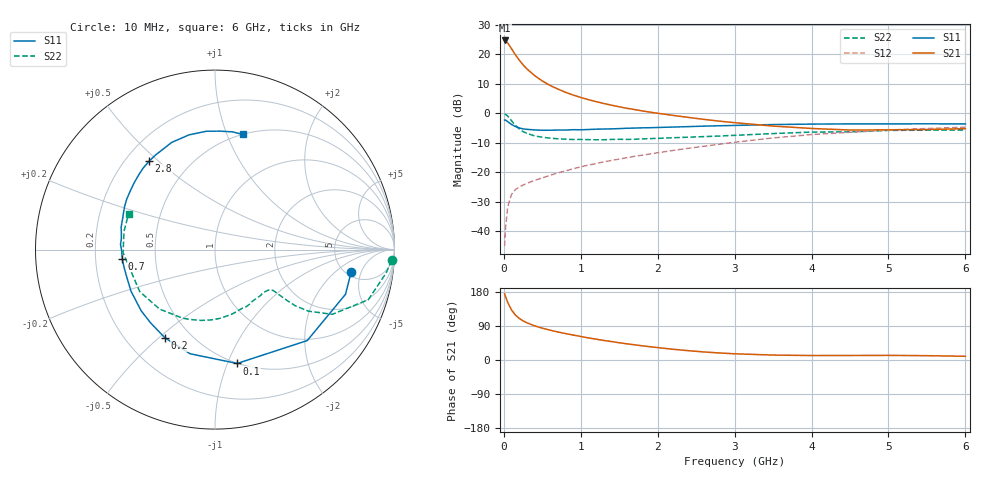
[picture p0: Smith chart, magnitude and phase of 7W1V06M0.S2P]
! Infineon Technologies  Discrete & RF Semiconductors
! BFS17W
! Si NPN RF Bipolar Junction Transistor in SOT323
! VCE = 1 V  IC = 6 mA
! Common Emitter S-Parameters:  August  1999
# GHz  S  MA  R  50
!  f  S11  S21  S12  S22
! GHz  MAG  ANG  MAG  ANG  MAG  ANG  MAG  ANG
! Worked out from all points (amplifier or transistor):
!   36 points, 10 MHz to 6 GHz, reference 50 ohm
!   highest |S21| = 24.7 dB at 10 MHz (marker M1)
!   |S21| within 3 dB of that: start of sweep to 104.5 MHz
!   unconditionally stable (mu >= 1): 454.1 MHz to end of sweep
!   at 250 MHz: K = 0.68, MSG = 20.4 dB, |S12| = -24.3 dB
!   at 1.4 GHz: K = 1.32, MAG = 6.0 dB, |S12| = -16.0 dB
!   at 6 GHz: K = 1.12, MAG = -2.4 dB, |S12| = -4.7 dB
!   S11 on the Smith chart (normalised r, x): 10 MHz: 5.55, -3.38; 100 MHz: 0.50, -1.08; 200 MHz: 0.36, -0.52; 700 MHz: 0.32, -0.04; 2.8 GHz: 0.29, +0.47; 6 GHz: 0.50, +1.14
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0.01  0.7689 -9.3  17.14 174.7  0.0056 84.1  0.986 -3.5
0.02  0.7686 -18.9  17 168.3  0.0107 84.6  0.962 -7.8
0.05  0.7218 -44.6  15.55 152.0  0.026 69.0  0.8987 -18.1
0.1  0.6462 -79.0  12.39 132.1  0.0423 55.9  0.7463 -28.9
0.15  0.5967 -103.4  9.805 118.7  0.051 48.7  0.6229 -33.4
0.2  0.5653 -119.5  7.955 109.8  0.0562 46.4  0.5445 -35.0
0.25  0.5435 -131.4  6.611 103.3  0.0607 44.5  0.4901 -35.2
0.3  0.5342 -140.4  5.644 98.2  0.065 45.0  0.4569 -35.2
0.4  0.5221 -153.7  4.349 90.1  0.073 46.3  0.4132 -35.1
0.5  0.515 -162.4  3.53 84.1  0.0804 48.8  0.3928 -35.2
0.6  0.5163 -169.1  2.969 78.8  0.0887 50.6  0.3788 -36.2
0.7  0.5194 -174.5  2.578 74.1  0.0976 52.4  0.3698 -38.1
0.9  0.5272 176.9  2.039 65.9  0.1146 54.5  0.3593 -42.6
1.1  0.5305 169.5  1.7 58.3  0.1326 55.9  0.3577 -48.3
1.3  0.5409 162.8  1.465 51.6  0.1504 56.7  0.3558 -54.9
1.6  0.5574 154.8  1.215 42.7  0.1765 57.2  0.3605 -65.1
2.2  0.5841 140.5  0.92 28.3  0.2346 57.2  0.385 -86.7
2.8  0.6142 126.7  0.736 18.6  0.2987 54.7  0.4115 -108.5
3.5  0.6441 112.0  0.607 13.0  0.3821 49.1  0.4529 -132.9
4.5  0.6612 94.1  0.52 11.9  0.4758 37.4  0.4839 -165.9
5.5  0.6631 81.5  0.531 11.4  0.552 26.4  0.517 168.6
6  0.6599 76.5  0.548 9.8  0.5824 21.1  0.5213 157.4
